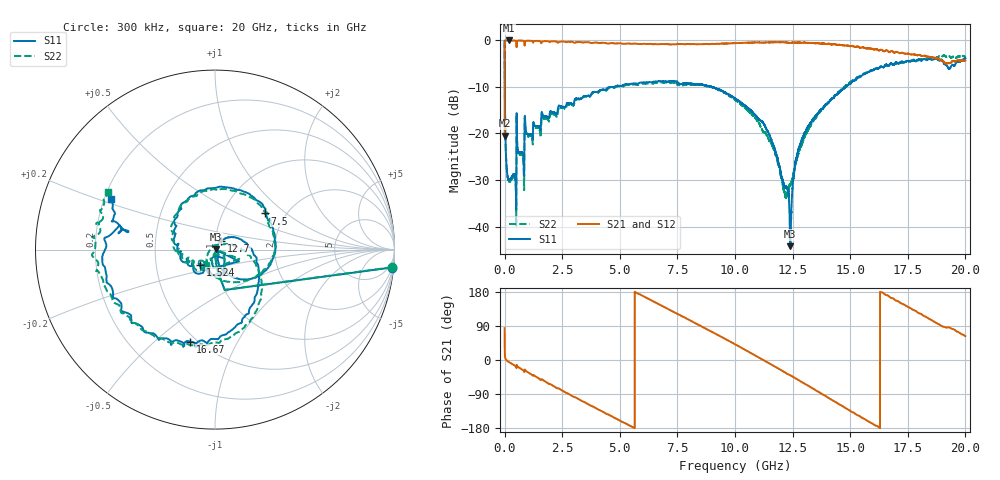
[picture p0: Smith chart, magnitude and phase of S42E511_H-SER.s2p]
! Created Wed Nov 25 22:19:42 2020
# khz S ma R 50
! 2 Port Network Data from SP1.SP block
! freq  magS11  angS11  magS21  angS21  magS12  angS12  magS22  angS22
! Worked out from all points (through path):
!   20001 points, 300 kHz to 20 GHz, reference 50 ohm
!   highest |S21| = -0.02 dB at 192.3 MHz (marker M1); lowest = -20.5 dB at 300 kHz (marker M2)
!   group delay of S21, straight-line fit = 92.2 ps
!   lowest |S11| = -44.2 dB at 12.4 GHz (marker M3), VSWR 1.01, Z = 50.6 + j0.214 ohm
!   |S11| at or under -10 dB: 9.477 MHz to 4.753 GHz (4.744 GHz wide, 199 % of centre); 4.754004 GHz to 4.758406 GHz (4.401 MHz wide, 0.0925 % of centre); 9.007 GHz to 14.8 GHz (5.793 GHz wide, 48.7 % of centre)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
!   |S22| runs from -39.8 to -0.1 dB; largest |S21 - S12| = 0.015
!   S11 on the Smith chart (normalised r, x): 300 kHz: 2, -20; 1.524 GHz: 0.84, -0.14; 7.5 GHz: 1.57, +0.72; 12.7 GHz: 1.06, +0.10; 16.67 GHz: 0.46, -0.66; 20 GHz: 0.23, +0.22
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300  0.9895 -5.8  0.09474 83.8  0.09442 83.7  0.9905 -5.7
110300  0.03731 -88.2  0.9967 -2.0  0.9967 -2.1  0.03688 -88.0
192300  0.03159 -92.4  0.9975 -5.5  0.9954 -5.5  0.03079 -92.6
413300  0.03656 -99.1  0.9959 -13.6  0.9956 -13.6  0.03456 -100.6
613300  0.06297 -107.7  0.9944 -19.6  0.9947 -19.6  0.05961 -108.3
961300  0.09983 -120.0  0.9881 -30.5  0.9897 -30.5  0.09501 -120.0
1524300  0.1169 -134.5  0.9831 -50.4  0.9831 -50.4  0.1076 -143.8
3334300  0.2362 157.9  0.9554 -107.6  0.9557 -107.6  0.2324 167.9
5019300  0.3242 111.3  0.929 -160.5  0.9293 -160.6  0.3185 110.7
6667300  0.3632 61.5  0.9087 148.1  0.9084 147.9  0.3504 56.8
7500300  0.3427 36.0  0.9181 122.1  0.9138 122.1  0.3298 29.8
8711300  0.3287 -7.8  0.9138 83.2  0.9148 83.2  0.3277 -5.6
1.00003e7  0.2385 -44.4  0.9328 41.6  0.9317 41.5  0.2299 -50.9
1.14043e7  0.1069 -72.1  0.9506 -5.7  0.9506 -5.8  0.09394 -117.4
1.21673e7  0.02664 -40.6  0.9533 -32.7  0.9516 -32.8  0.02259 159.0
1.24033e7  0.006159 20.1  0.9396 -40.4  0.9377 -40.6  0.02818 59.3
1.26953e7  0.05779 54.3  0.9457 -50.8  0.9464 -50.9  0.05398 33.4
1.33343e7  0.1346 28.6  0.9381 -73.7  0.9374 -73.9  0.1289 6.2
1.50923e7  0.3624 -52.8  0.8679 -137.6  0.8702 -137.4  0.3692 -45.9
1.66673e7  0.5305 -105.1  0.7541 168.9  0.758 168.1  0.5434 -99.7
1.82413e7  0.6261 -155.1  0.6831 115.2  0.6782 115.8  0.6329 -151.8
2e7  0.6412 154.0  0.6054 62.8  0.6044 63.0  0.6818 151.5
